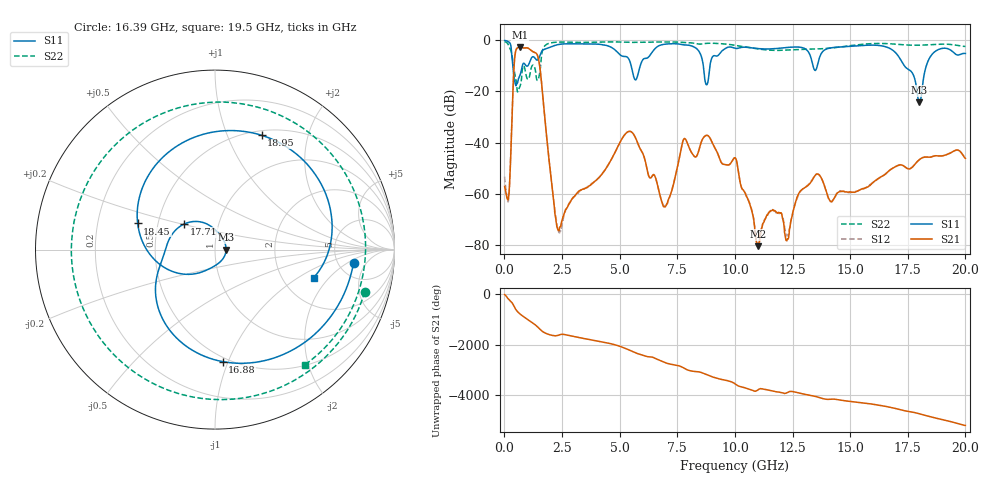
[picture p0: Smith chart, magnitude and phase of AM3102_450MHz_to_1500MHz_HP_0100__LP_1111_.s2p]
!Agilent Technologies,E8364B,MY43040894,A.07.50.67
!Agilent E8364B: A.07.50.67
!Date: Thursday, January 11, 2018 05:38:59
!Correction: S11(Full 2 Port(1,2))
!S21(Full 2 Port(1,2))
!S12(Full 2 Port(1,2))
!S22(Full 2 Port(1,2))
!S2P File: Measurements: S11, S21, S12, S22:
# Hz S  dB  R 50
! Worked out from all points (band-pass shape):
!   1601 points, 10 MHz to 20 GHz, reference 50 ohm
!   highest |S21| = -2.70 dB at 672.2 MHz (marker M1); lowest = -80.5 dB at 11 GHz (marker M2)
!   |S21| within 3 dB of the highest: 462.8 MHz to 1.426 GHz (963.3 MHz wide, 102 % of centre)
!   lowest |S11| = -24.2 dB at 18 GHz (marker M3), VSWR 1.13, Z = 56.6 - j0.0129 ohm
!   |S11| at or under -10 dB: 367.3 MHz to 777.8 MHz (410.5 MHz wide, 71.7 % of centre); 5.502 GHz to 5.893 GHz (391.1 MHz wide, 6.87 % of centre); 17.36 GHz to 18.3 GHz (947.7 MHz wide, 5.32 % of centre)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
!   |S22| runs from -20.2 to -0.5 dB; largest |S21 - S12| = 0.0015
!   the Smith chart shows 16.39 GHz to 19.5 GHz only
!   S11 on the Smith chart (normalised r, x): 16.39 GHz: 6.97, -2.54; 16.88 GHz: 0.47, -0.96; 17.71 GHz: 0.68, +0.21; 18.45 GHz: 0.38, +0.14; 18.95 GHz: 0.55, +1.34; 19.5 GHz: 2.97, -1.37
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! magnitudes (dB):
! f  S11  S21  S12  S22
! 10 MHz  -0.1  -57.2  -53.3  -0.5
! 184.9 MHz  -0.6  -61.2  -62.1  -2.0
! 447.3 MHz  -15.9  -7.0  -7.0  -12.9
! 672.2 MHz  -13.8  -2.7  -2.7  -18.2
! 1.472 GHz  -7.4  -7.0  -7.0  -15.2
! 2.346 GHz  -1.7  -74.4  -74.7  -0.7
! 3.346 GHz  -1.4  -58.5  -58.3  -0.8
! 5.42 GHz  -7.7  -35.6  -35.6  -0.8
! 6.682 GHz  -2.2  -58.0  -58.1  -0.7
! 7.819 GHz  -1.8  -38.4  -38.5  -0.9
! 10.01 GHz  -3.1  -45.9  -46.0  -2.0
! 11 GHz  -3.2  -80.5  -80.1  -3.4
! 13.34 GHz  -8.2  -54.9  -54.7  -3.4
! 16.39 GHz  -2.2  -53.1  -53.1  -1.2
! 16.68 GHz  -3.0  -51.1  -51.1  -1.3
! 16.88 GHz  -4.1  -49.9  -49.8  -1.5
! 17.71 GHz  -13.0  -49.5  -49.4  -1.9
! 18 GHz  -24.2  -46.7  -46.7  -1.9
! 18.45 GHz  -6.8  -45.7  -45.7  -1.7
! 18.95 GHz  -3.2  -45.3  -45.3  -1.5
! 19.5 GHz  -4.9  -43.3  -43.3  -1.8
! 20 GHz  -5.1  -46.2  -46.0  -2.4
